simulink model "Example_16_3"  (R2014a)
settings: Solver=ode45  StartTime=0.0  StopTime=10.0  RelTol=1e-3

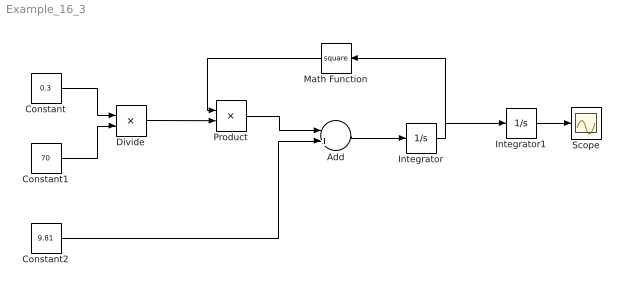
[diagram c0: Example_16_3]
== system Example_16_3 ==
  Add : Sum  Inputs=-+
  Constant : Constant  Value=0.3
  Constant1 : Constant  Value=70
  Constant2 : Constant  Value=9.81
  Divide : Product  Inputs=*/
  Integrator : Integrator
  Integrator1 : Integrator
  Math Function : Math  Operator=square
  Product : Product
  Scope : Scope
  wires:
  Constant/1 -> Divide/1
  Constant1/1 -> Divide/2
  Divide/1 -> Product/2
  Math Function/1 -> Product/1
  Product/1 -> Add/1
  Constant2/1 -> Add/2
  Add/1 -> Integrator/1
  Integrator/1 -> Math Function/1, Integrator1/1
  Integrator1/1 -> Scope/1
